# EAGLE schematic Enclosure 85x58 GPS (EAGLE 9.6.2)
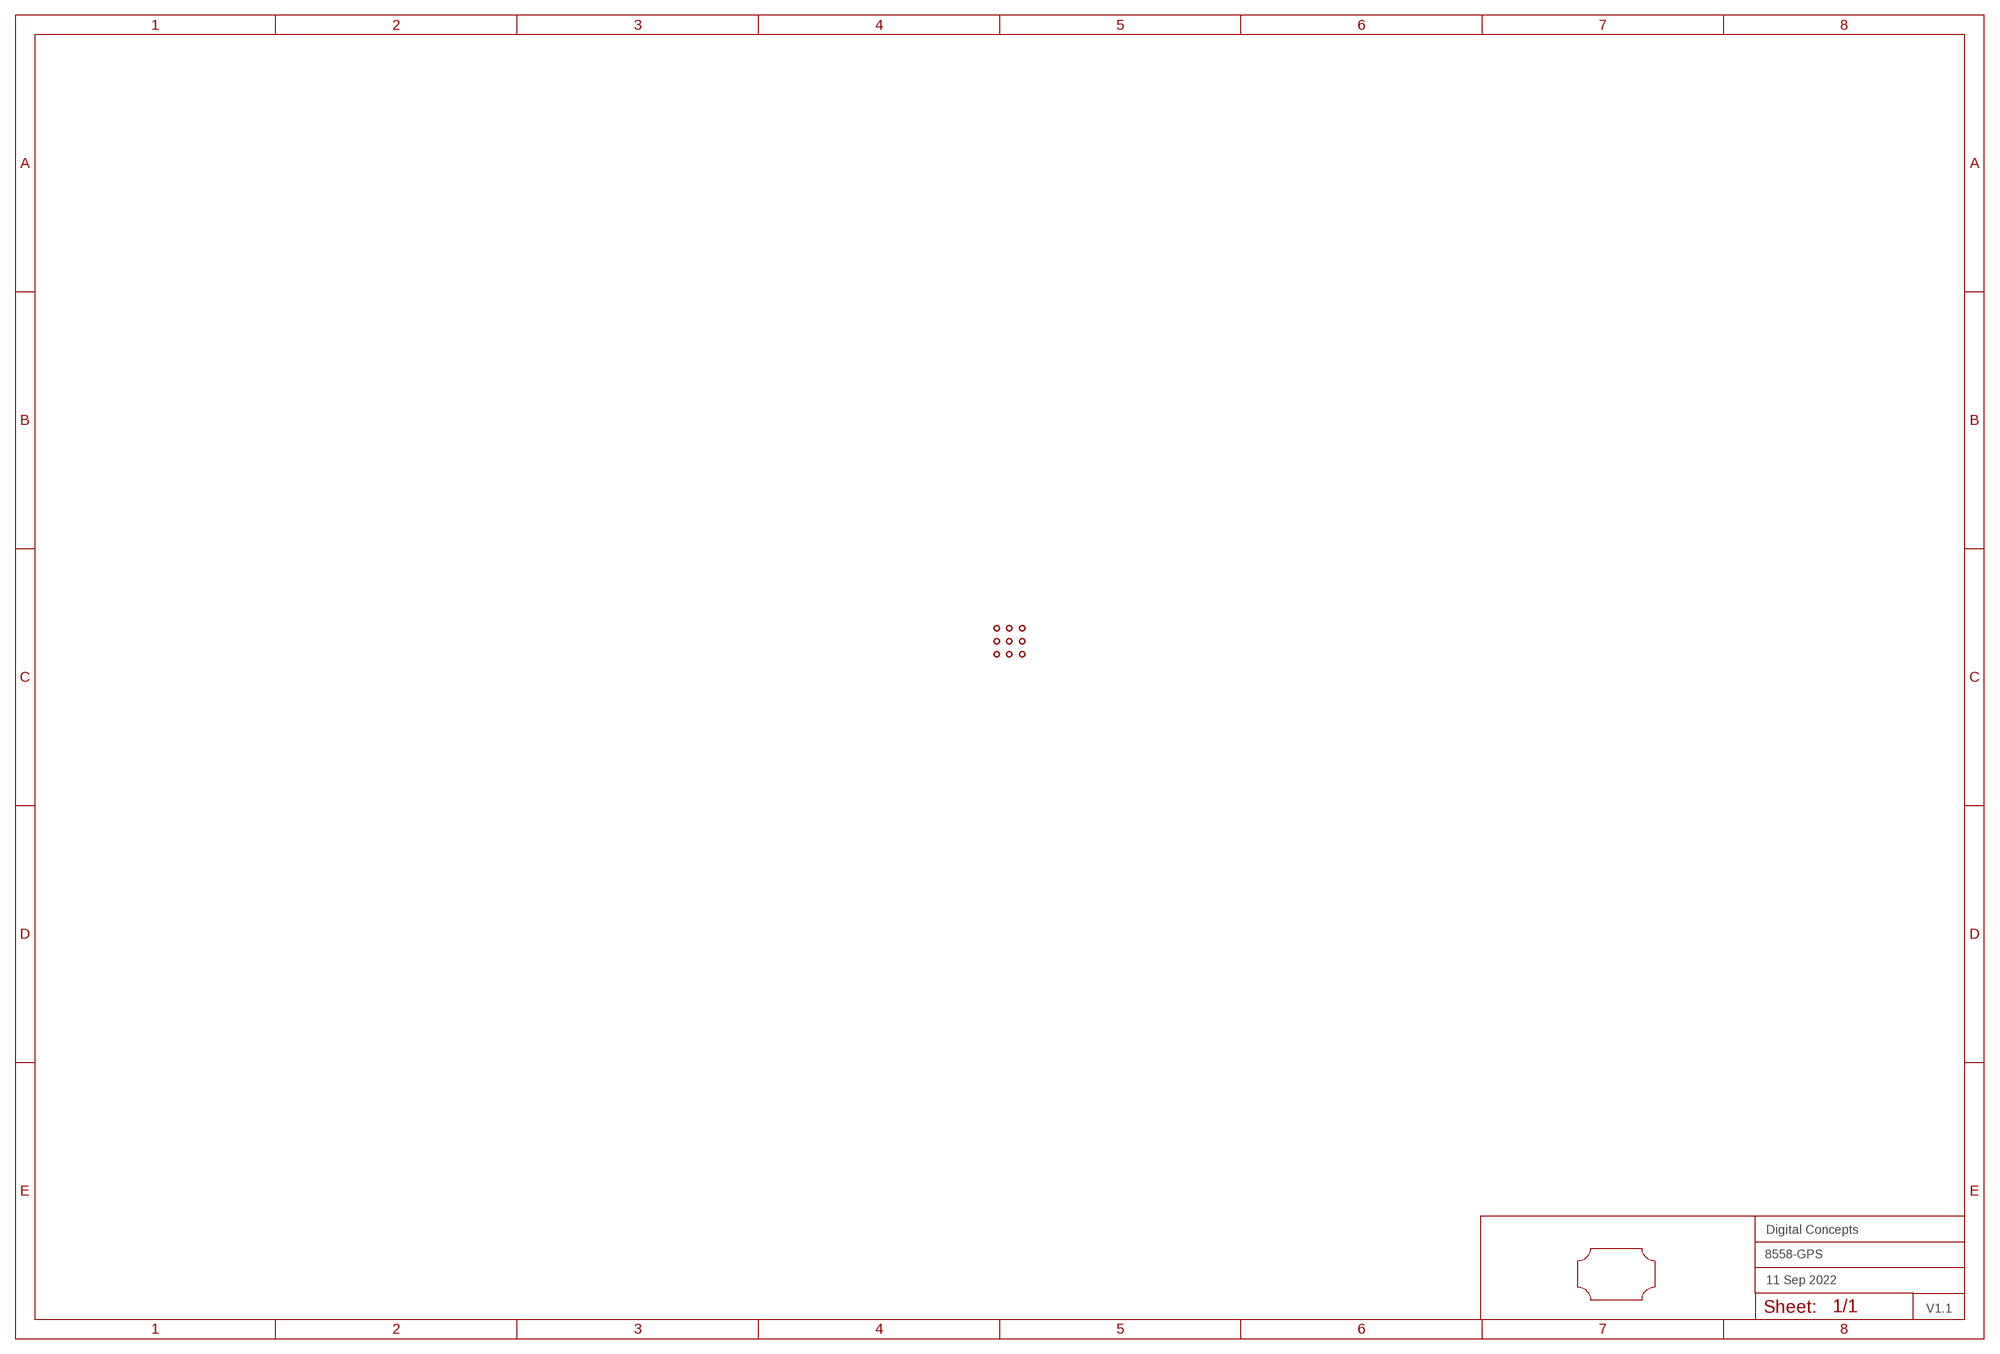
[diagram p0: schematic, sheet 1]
FRAME2 (A3L-LOC): DATE: 11 Sep 2022; OWNER: Digital Concepts; TITLE: 8558-GPS; VERSION: V1.1

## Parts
U$1  PROTO-28X18-GPS  [PROTO-28X18-GPS]
U$2  PCB-OUTLINE-A-85X58  [PROTO-28X18-OUTLINE-A]

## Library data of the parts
U$1 = digitalconcepts:PROTO-28X18-GPS: 28 x 18 Prototyping board to fit an 85 x 58 enclosure
U$2 = digitalconcepts:PCB-OUTLINE-A-85X58: PCB outline with hole blank for 85 x 58 enclosure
